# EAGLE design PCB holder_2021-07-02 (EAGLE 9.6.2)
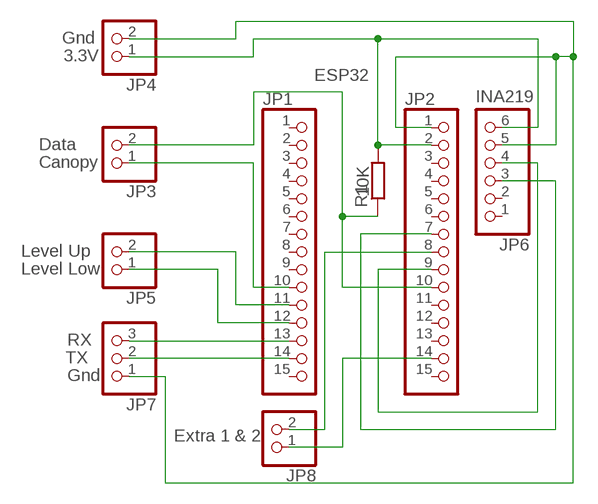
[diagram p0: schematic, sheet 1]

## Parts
JP1  PINHD-1X15  [1X15]
JP2  PINHD-1X15  [1X15]
JP3  PINHD-1X2/90  [1X02/90]
JP4  PINHD-1X2/90  [1X02/90]
JP5  PINHD-1X2/90  [1X02/90]
JP6  PINHD-1X6  [1X06]
JP7  PINHD-1X3/90  [1X03/90]
JP8  PINHD-1X2/90  [1X02/90]
R1  10K  R-EU_0207/10  [0207/10]

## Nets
N$1: JP2.2 JP4.1 JP6.6 R1.2
N$2: JP2.1 JP4.2 JP6.5 JP7.1
N$3: JP2.7 JP6.3
N$4: JP2.9 JP6.4
N$5: JP2.10 JP3.2 R1.1
N$6: JP1.14 JP7.2
N$7: JP1.13 JP7.3
N$8: JP2.14 JP8.1
N$9: JP1.12 JP5.1
N$10: JP1.11 JP5.2
N$11: JP1.10 JP3.1
N$12: JP2.8 JP8.2
Unconnected: JP1.1 JP1.2 JP1.3 JP1.4 JP1.5 JP1.6 JP1.7 JP1.8 JP1.9 JP1.15 JP2.3 JP2.4 JP2.5 JP2.6 JP2.11 JP2.12 JP2.13 JP2.15 JP6.1 JP6.2

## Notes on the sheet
- Gnd
- 3.3V
- ESP32
- INA219
- Data
- Canopy
- Level Up
- Level Low
- RX
- TX
- Gnd
- Extra 1 & 2

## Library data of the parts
JP1 JP2 = pinhead:PINHD-1X15: PIN HEADER
JP3-JP5 JP8 = pinhead:PINHD-1X2: PIN HEADER
JP6 = pinhead:PINHD-1X6: PIN HEADER
JP7 = pinhead:PINHD-1X3: PIN HEADER
R1 = rcl:R-EU_: RESISTOR, European symbol; SPICEPREFIX: R

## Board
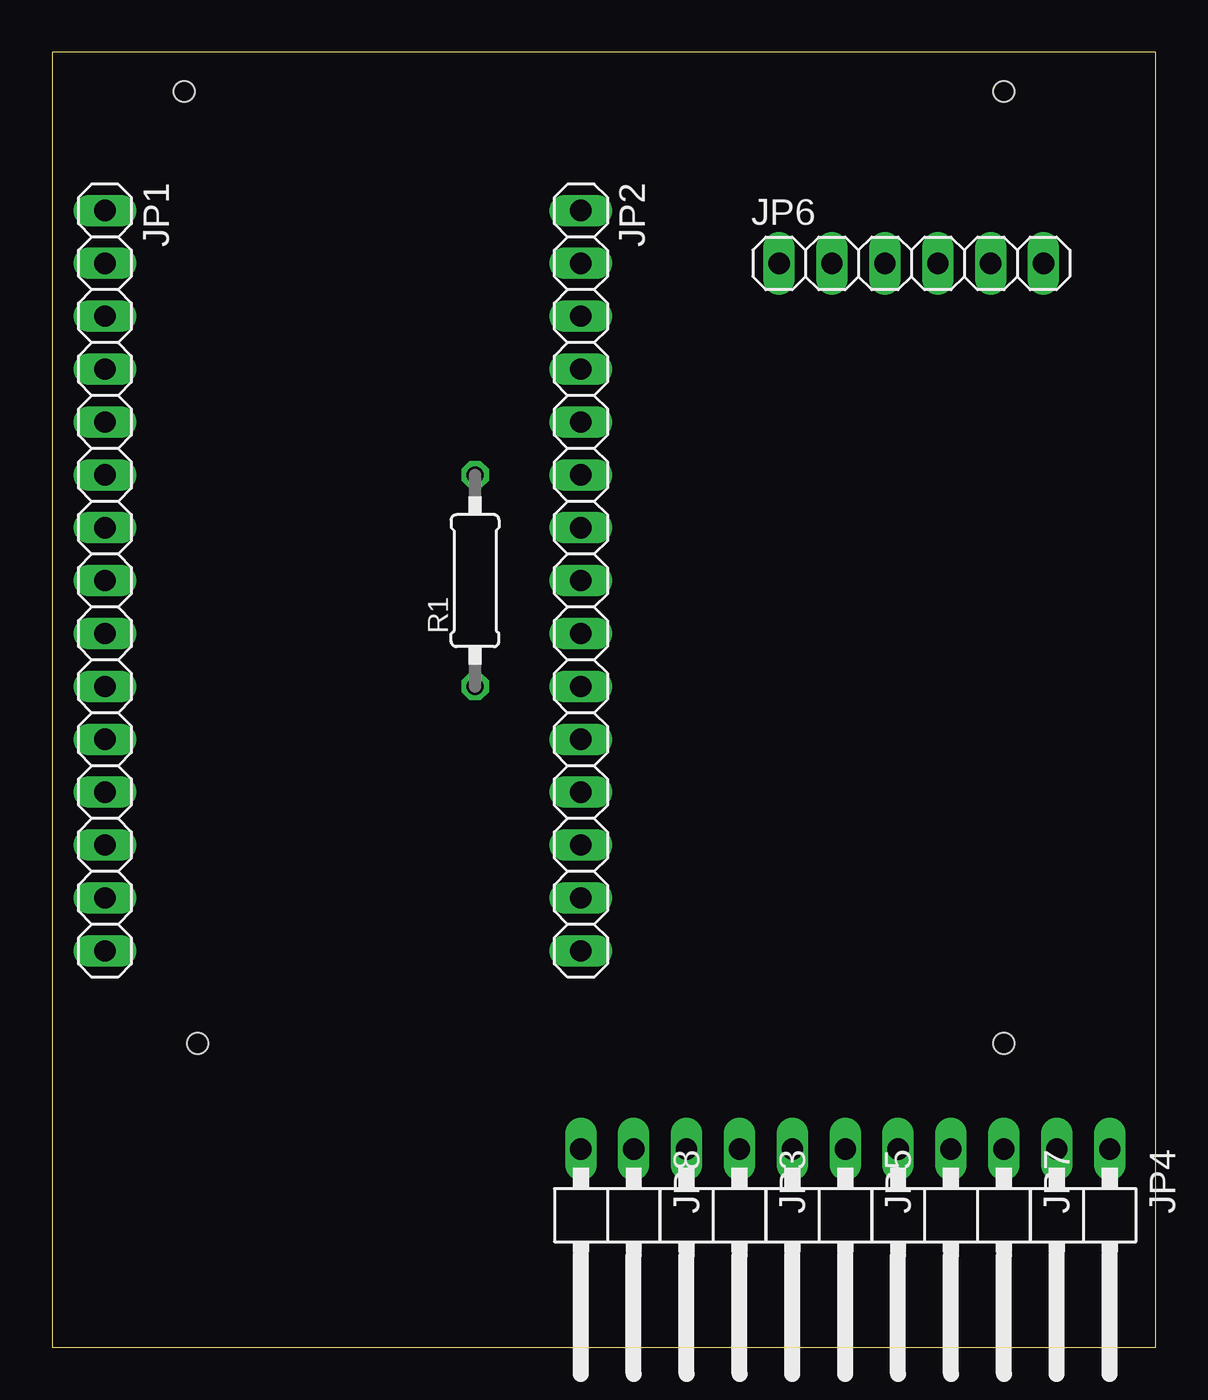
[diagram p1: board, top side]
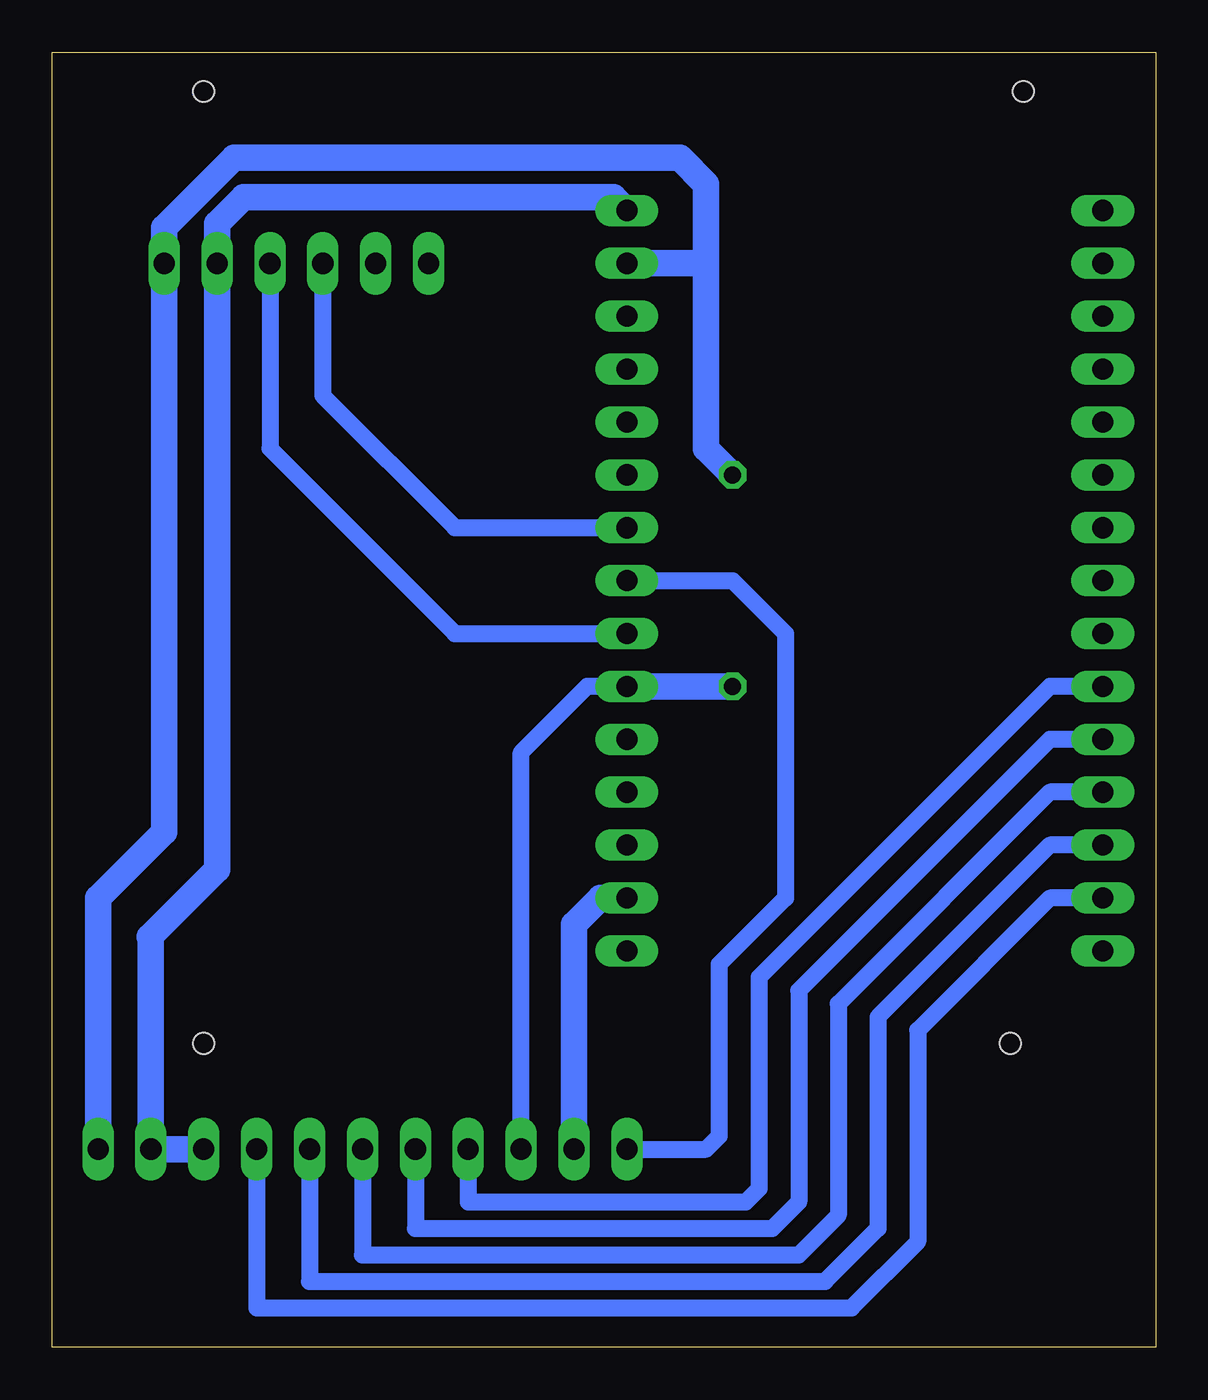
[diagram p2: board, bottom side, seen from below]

Size 53.01 x 62.22 mm. Coordinates in mm from the lower left corner, seen from the top.
Outline: 0,0 53.01,0 53.01,62.22 0,62.22 0,0
Copper layers (1*16): Top 0.035mm / dielectric 1.5mm / Bottom 0.035mm
Design rules "default": minimum track width 6mil, minimum drill 0.35mm, track to track 6mil, track to pad 6mil, pad to pad 6mil, via to via 6mil, smd to smd 6mil, copper to edge 40mil, drill to drill 6mil, minimum pad ring 10mil, minimum via ring 8mil, stop-mask expansion 4mil, vias tented up to drill 0mil, thermal gap 10mil
Holes 1 mm at 45.72,14.61 6.35,60.33 45.72,60.33 6.99,14.61

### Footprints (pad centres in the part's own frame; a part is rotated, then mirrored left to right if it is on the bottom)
1X15 = drill 1.016 long: 1 -17.78,0; 2 -15.24,0; 3 -12.7,0; 4 -10.16,0; 5 -7.62,0; 6 -5.08,0; 7 -2.54,0; 8 0,0; 9 2.54,0; 10 5.08,0; 11 7.62,0; 12 10.16,0; 13 12.7,0; 14 15.24,0; 15 17.78,0
1X02/90 = drill 1.016 long: 1 -1.27,-3.81; 2 1.27,-3.81
1X06 = drill 1.016 long: 1 -6.35,0; 2 -3.81,0; 3 -1.27,0; 4 1.27,0; 5 3.81,0; 6 6.35,0
1X03/90 = drill 1.016 long: 1 -2.54,-3.81; 2 0,-3.81; 3 2.54,-3.81
0207/10 = drill 0.813 octagon: 1 -5.08,0; 2 5.08,0

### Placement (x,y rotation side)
JP1  2.54,36.83 270 top
JP2  25.4,36.83 270 top
JP3  31.75,5.71 180 top
JP4  49.53,5.71 180 top
JP5  36.83,5.71 180 top
JP6  41.27,52.07 0 top
JP7  43.18,5.71 180 top
JP8  26.67,5.71 180 top
R1  20.32,36.83 90 top

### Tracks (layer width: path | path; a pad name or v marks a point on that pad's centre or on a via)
N$1
  Bottom 1.27: JP2.2 21.59,52.07 | 21.59,52.07 21.59,43.18 R1.2 | 21.59,52.07 21.59,55.88 22.86,57.15 44.27,57.15 47.62,53.8 JP6.6 47.62,24.77 50.8,21.59 JP4.1
N$2
  Bottom 0.813: 48.26,19.67 48.31,19.72
  Bottom 1.27: JP2.1 26.04,55.24 43.81,55.24 45.09,53.98 JP6.5 45.09,22.95 48.31,19.72 | 48.26,19.67 JP4.2 JP7.1
N$3
  Bottom 0.813: JP2.7 33.66,39.37 40.01,45.72 JP6.3
N$4
  Bottom 0.813: JP2.9 33.66,34.29 42.55,43.18 JP6.4
N$5
  Bottom 0.813: JP3.2 30.48,28.57 27.3,31.75 JP2.10
  Bottom 1.27: R1.1 JP2.10
N$6
  Bottom 0.813: JP7.2 43.18,1.91 14.61,1.91 11.43,5.08 11.43,15.24 5.08,21.59 JP1.14
N$7
  Bottom 0.813: JP7.3 40.64,3.17 15.88,3.17 13.34,5.71 13.34,15.88 5.08,24.13 JP1.13
N$8
  Bottom 1.27: JP2.14 26.67,21.59 27.94,20.32 JP8.1
N$9
  Bottom 0.813: JP5.1 38.1,4.45 17.14,4.45 15.24,6.35 15.24,16.51 5.08,26.67 JP1.12
N$10
  Bottom 0.813: JP5.2 35.56,5.71 18.41,5.71 17.14,6.99 17.14,17.14 5.08,29.21 JP1.11
N$11
  Bottom 0.813: JP3.1 33.02,6.99 19.68,6.99 19.05,7.62 19.05,17.78 5.08,31.75 JP1.10
N$12
  Bottom 0.813: JP8.2 21.59,9.53 20.95,10.16 20.95,18.41 17.78,21.59 17.78,34.29 20.32,36.83 JP2.8

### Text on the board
tDocu: ESP32 | INA219 | Ex1 | Ex2 | Data | Canopy | Level Up | Level Low | RX | TX | Gnd | 3.3V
